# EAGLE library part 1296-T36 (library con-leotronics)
1.27mm SINGLE ROW FEMALE SOCKET Source: http://www.leotronics.co.uk/Conexcon/Data%20Sheets/sec.%20A/1296ing.pdf
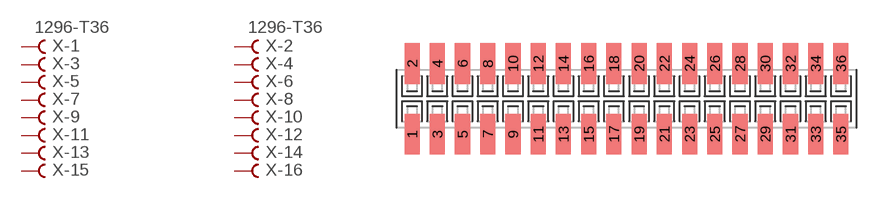
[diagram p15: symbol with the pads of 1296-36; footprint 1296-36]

Designator prefix X; gates -1=FVAL -2=FVAL -3=F -4=F -5=F -6=F -7=F -8=F -9=F -10=F -11=F -12=F -13=F -14=F -15=F -16=F -17=F -18=F -19=F -20=F -21=F -22=F -23=F -24=F -25=F -26=F -27=F -28=F -29=F -30=F -31=F -32=F -33=F -34=F -35=F -36=F

## 1296-T36 (OC_FARNELL: unknown; OC_NEWARK: unknown)  [1296-36]
1  -1:B  pas
2  -2:B  pas
3  -3:B  pas
4  -4:B  pas
5  -5:B  pas
6  -6:B  pas
7  -7:B  pas
8  -8:B  pas
9  -9:B  pas
10  -10:B  pas
11  -11:B  pas
12  -12:B  pas
13  -13:B  pas
14  -14:B  pas
15  -15:B  pas
16  -16:B  pas
17  -17:B  pas
18  -18:B  pas
19  -19:B  pas
20  -20:B  pas
21  -21:B  pas
22  -22:B  pas
23  -23:B  pas
24  -24:B  pas
25  -25:B  pas
26  -26:B  pas
27  -27:B  pas
28  -28:B  pas
29  -29:B  pas
30  -30:B  pas
31  -31:B  pas
32  -32:B  pas
33  -33:B  pas
34  -34:B  pas
35  -35:B  pas
36  -36:B  pas

## Footprint 1296-36 (pad centres in mm)
1.27mm SINGLE ROW FEMALE SOCKET Source: http://www.leotronics.co.uk/Conexcon/Data%20Sheets/sec.%20A/1296ing.pdf
smd 0.76 x 2.05: 1 -10.795,-1.78; 2 -10.795,1.78; 3 -9.525,-1.78; 4 -9.525,1.78; 5 -8.255,-1.78; 6 -8.255,1.78; 7 -6.985,-1.78; 8 -6.985,1.78; 9 -5.715,-1.78; 10 -5.715,1.78; 11 -4.445,-1.78; 12 -4.445,1.78; 13 -3.175,-1.78; 14 -3.175,1.78; 15 -1.905,-1.78; 16 -1.905,1.78; 17 -0.635,-1.78; 18 -0.635,1.78; 19 0.635,-1.78; 20 0.635,1.78; 21 1.905,-1.78; 22 1.905,1.78; 23 3.175,-1.78; 24 3.175,1.78; 25 4.445,-1.78; 26 4.445,1.78; 27 5.715,-1.78; 28 5.715,1.78; 29 6.985,-1.78; 30 6.985,1.78; 31 8.255,-1.78; 32 8.255,1.78; 33 9.525,-1.78; 34 9.525,1.78; 35 10.795,-1.78; 36 10.795,1.78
